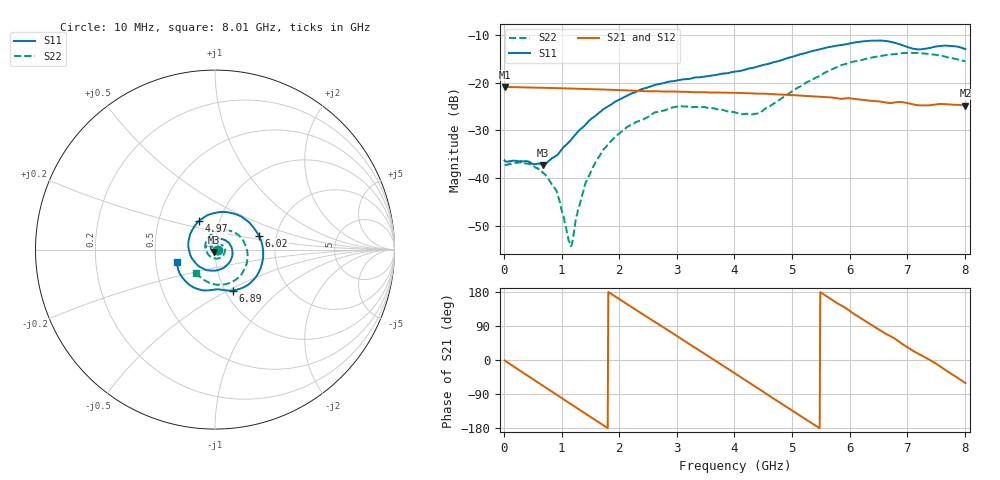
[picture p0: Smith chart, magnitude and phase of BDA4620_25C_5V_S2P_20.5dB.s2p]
!Agilent Technologies,E5071B,MY42404982,A.09.10
!Date: Wed May 06 09:02:44 2026
!Data & Calibration Information:
!Freq	S11:SOLT2(ON)	S21:SOLT2(ON)	S12:SOLT2(ON)	S22:SOLT2(ON)
# Hz S RI R 50
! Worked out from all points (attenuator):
!   801 points, 10 MHz to 8.01 GHz, reference 50 ohm
!   highest |S21| = -20.91 dB at 10 MHz (marker M1); lowest = -24.8 dB at 8.01 GHz (marker M2)
!   lowest |S11| = -37.3 dB at 680 MHz (marker M3), VSWR 1.03, Z = 49.6 - j1.31 ohm
!   |S11| at or under -10 dB: start of sweep to end of sweep
!   |S22| runs from -54.2 to -13.8 dB; largest |S21 - S12| = 0.00041
!   S11 on the Smith chart (normalised r, x): 10 MHz: 1.03, -0.00; 4.97 GHz: 0.80, +0.27; 6.02 GHz: 1.62, +0.26; 6.89 GHz: 1.08, -0.53; 8.01 GHz: 0.65, -0.10
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1e7  0.0153 -0.00107  0.0901 -0.0019  0.0902 -0.00195  0.0137 -0.000474
4.2e8  0.00809 -0.0126  0.0653 -0.0599  0.0655 -0.0602  0.0133 -0.00488
6.8e8  -0.00373 -0.0132  0.0322 -0.0819  0.0322 -0.0821  0.00907 -0.00677
9.2e8  -0.0161 -0.00649  -0.00376 -0.0872  -0.00387 -0.0873  0.0035 -0.00621
1.15e9  -0.0233 0.00809  -0.0371 -0.0782  -0.0372 -0.0783  -0.00158 -0.00118
1.19e9  -0.0239 0.0113  -0.0423 -0.0753  -0.0424 -0.0753  -0.00223 0.00011
1.35e9  -0.0231 0.0241  -0.0608 -0.0604  -0.0609 -0.0606  -0.00384 0.00514
1.53e9  -0.0161 0.0393  -0.0758 -0.0388  -0.0759 -0.0387  -0.00347 0.0119
1.77e9  0.00307 0.0546  -0.0841 -0.00504  -0.0843 -0.00501  0.000907 0.0213
2.14e9  0.0467 0.0564  -0.0695 0.0452  -0.0696 0.0454  0.0172 0.0297
2.68e9  0.0961 0.000132  -0.00653 0.0806  -0.00642 0.0808  0.0454 0.0191
3.47e9  0.021 -0.1133  0.0755 0.0239  0.0757 0.0239  0.0405 -0.0379
4.01e9  -0.0958 -0.0878  0.0635 -0.0454  0.0636 -0.0455  -0.0119 -0.0474
4.42e9  -0.1478 0.0093  0.0188 -0.0742  0.0186 -0.0743  -0.046 -0.0125
4.97e9  -0.0871 0.1611  -0.0477 -0.0565  -0.0479 -0.0565  -0.0356 0.0702
5.35e9  0.0365 0.2099  -0.0699 -0.0156  -0.07 -0.0156  0.0234 0.1041
6.02e9  0.2454 0.0755  -0.0416 0.0543  -0.0417 0.0544  0.1522 0.0581
6.35e9  0.264 -0.0684  -0.00619 0.0642  -0.00612 0.0643  0.1797 -0.0115
6.68e9  0.1814 -0.1979  0.0258 0.0554  0.0259 0.0555  0.1714 -0.092
6.89e9  0.0981 -0.2284  0.0442 0.0443  0.0443 0.0444  0.1468 -0.1391
7.56e9  -0.0979 -0.219  0.0573 -0.0162  0.0574 -0.0161  -0.0153 -0.1904
8.01e9  -0.2109 -0.0716  0.028 -0.0499  0.0282 -0.05  -0.1059 -0.1278
